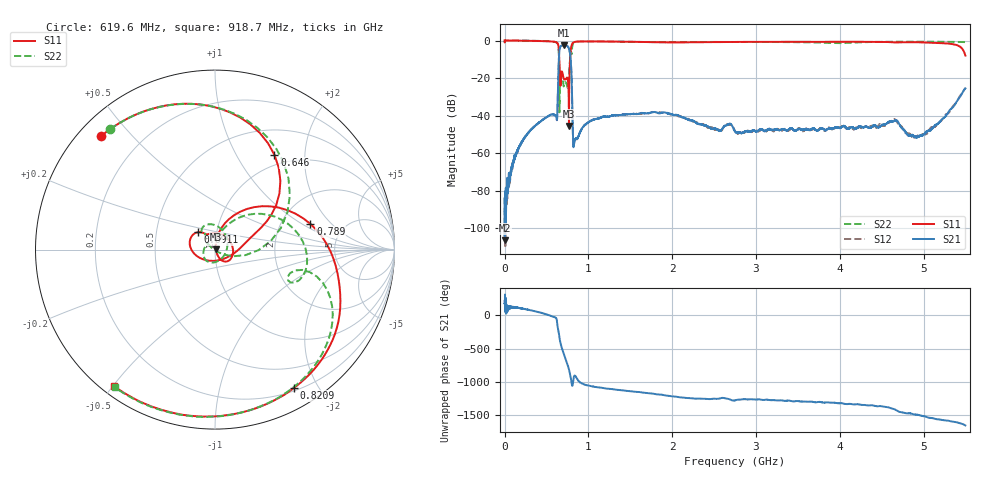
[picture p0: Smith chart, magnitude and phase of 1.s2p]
!Keysight Technologies,N5232A,MY52221221,A.10.65.11
!Date: Friday, July 07, 2023 15:39:58
!Correction: S11(Full 2 Port(1,4))
!S41(Full 2 Port(1,4))
!S14(Full 2 Port(1,4))
!S44(Full 2 Port(1,4))
!S2P File: Measurements: S11, S41, S14, S44:
# Hz S  RI  R 50
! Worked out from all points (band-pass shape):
!   5001 points, 300 kHz to 5.5 GHz, reference 50 ohm
!   highest |S21| = -2.42 dB at 705.4 MHz (marker M1); lowest = -106.4 dB at 2.5 MHz (marker M2)
!   |S21| within 3 dB of the highest: 653.9 MHz to 775.5 MHz (121.6 MHz wide, 17 % of centre)
!   lowest |S11| = -45.5 dB at 768.1 MHz (marker M3), VSWR 1.01, Z = 50.5 + j0.0675 ohm
!   |S11| at or under -10 dB: 652.9 MHz to 781.1 MHz (128.2 MHz wide, 17.9 % of centre)
!   |S22| runs from -38.3 to 0.0 dB; largest |S21 - S12| = 0.0032
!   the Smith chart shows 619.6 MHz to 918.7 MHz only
!   S11 on the Smith chart (normalised r, x): 619.6 MHz: 0.06, +0.41; 646 MHz: 0.84, +1.45; 691.1 MHz: 0.81, +0.16; 789 MHz: 2.91, +1.19; 820.9 MHz: 0.24, -1.70; 918.7 MHz: 0.03, -0.50
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300000  1.003 -0.00435  -5.99e-05 5.32e-06  -5.21e-05 4.15e-05  1.003 -0.00734
2499880  0.9202 0.1173  -2.94e-06 -3.78e-06  4.44e-06 3.61e-06  0.9325 0.1213
3.555806e8  -0.1645 -0.9698  0.00223 0.0046  0.00216 0.00458  -0.1734 -0.9694
5.524699e8  -0.9301 -0.1991  0.0105 -0.00137  0.0104 -0.00149  -0.9353 -0.1766
6.195662e8  -0.6347 0.6322  0.00549 -0.00645  0.00558 -0.00644  -0.5834 0.6718
6.459648e8  0.3314 0.5274  -0.0777 0.2375  -0.0775 0.2365  0.4173 0.3019
6.910623e8  -0.0944 0.0967  -0.7085 -0.2334  -0.7092 -0.2335  0.0489 0.0969
7.053615e8  -0.0471 0.0852  -0.6263 0.425  -0.6255 0.4253  0.0457 -0.0392
7.394597e8  0.1006 -0.00147  0.6575 0.3262  0.6573 0.3275  -0.0647 -0.0275
7.680581e8  0.00527 0.000668  -0.0253 -0.6176  -0.0262 -0.6173  0.0365 0.1048
7.88957e8  0.5316 0.143  -0.2376 0.1669  -0.237 0.1668  0.5048 0.00496
8.208552e8  0.4407 -0.77  -0.000528 0.00141  -0.000562 0.00141  0.5226 -0.6863
8.42854e8  0.0868 -0.9194  -0.00227 0.000471  -0.0023 0.000567  0.143 -0.909
9.1765e8  -0.558 -0.7646  0.0024 0.0036  0.00237 0.00356  -0.552 -0.7715
9.187499e8  -0.5637 -0.7605  0.00244 0.00356  0.00248 0.00357  -0.5574 -0.7677
1.206934e9  -0.9328 0.1319  0.00864 -0.00364  0.00845 -0.0035  -0.9321 0.1442
1.8339e9  -0.181 0.8801  -0.00449 -0.0108  -0.00402 -0.0111  -0.1713 0.8887
2.75015e9  0.8076 0.4318  -0.00351 0.00132  -0.00358 0.0017  0.8216 0.4036
3.6675e9  0.6963 -0.6073  -0.00332 0.00294  -0.0031 0.00275  0.6627 -0.5936
4.58375e9  -0.3698 -0.8329  0.0042 0.00538  0.00407 0.00516  -0.2525 -0.8922
4.983028e9  -0.7616 -0.4697  0.000809 -0.00286  0.000806 -0.00296  -0.699 -0.6152
5.5e9  -0.2787 0.2835  -0.0409 0.034  -0.0439 0.0331  -0.9048 0.0895
